FUNCTION_BLOCK Preset_Encoder_DUT

VAR_IN_OUT
    SD_SMD_IO: DUT_AMCI_Stepper;
END_VAR	

VAR_INPUT
	FB_Target_Position: DINT;
	FB_Save_In_Flash_0_no_1_yes: UINT;
    		
END_VAR

VAR_OUTPUT
	Enable: BOOL :=FALSE;
	Error: BOOL :=TRUE;
END_VAR

VAR	
	I_Command_Word_1: UINT;
		
END_VAR

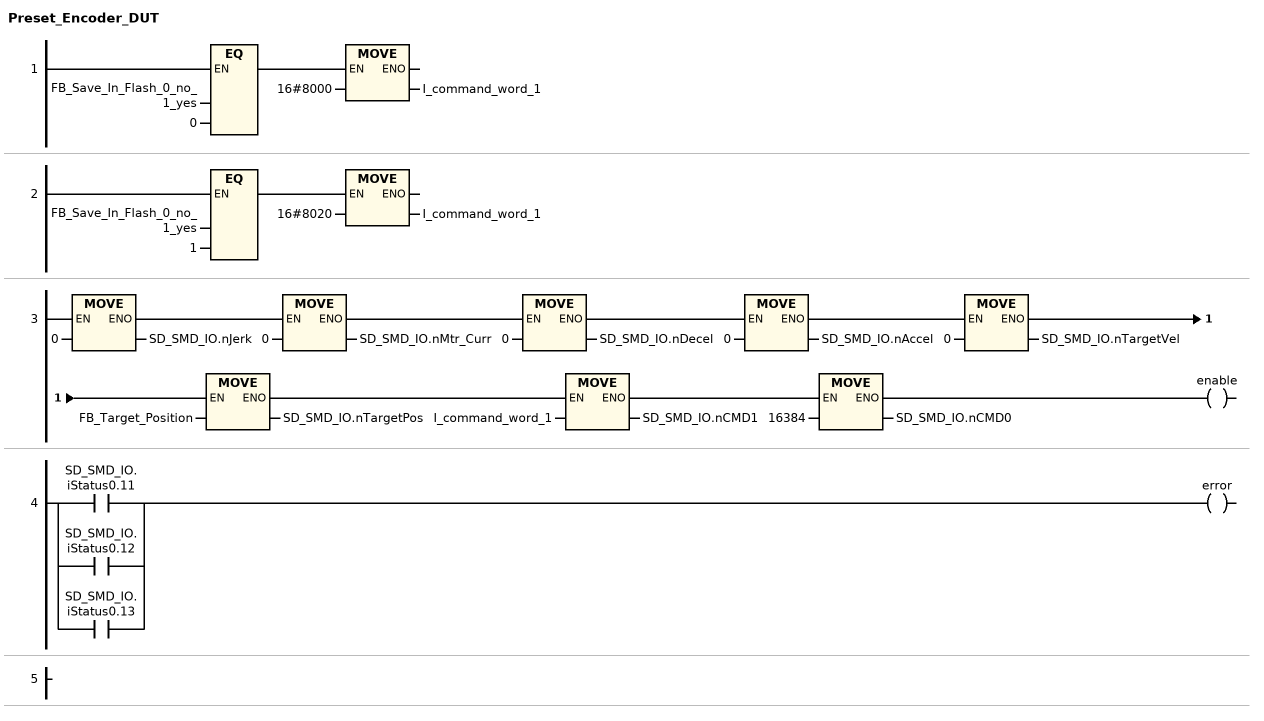
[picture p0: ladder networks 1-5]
// NETWORK 1
IF FB_Save_In_Flash_0_no_1_yes = 0 THEN I_command_word_1 := 16#8000; END_IF

// NETWORK 2
IF FB_Save_In_Flash_0_no_1_yes = 1 THEN I_command_word_1 := 16#8020; END_IF

// NETWORK 3
SD_SMD_IO.nJerk := 0;
SD_SMD_IO.nMtr_Curr := 0;
SD_SMD_IO.nDecel := 0;
SD_SMD_IO.nAccel := 0;
SD_SMD_IO.nTargetVel := 0;
SD_SMD_IO.nTargetPos := FB_Target_Position;
SD_SMD_IO.nCMD1 := I_command_word_1;
SD_SMD_IO.nCMD0 := 16384;
enable := TRUE;

// NETWORK 4
error := SD_SMD_IO.iStatus0.11 OR SD_SMD_IO.iStatus0.12 OR SD_SMD_IO.iStatus0.13;

// NETWORK 5

END_FUNCTION_BLOCK
